| TEXAS INSTRUMENTS INCORPORATED
| Standard Linear and Logic Group
| IBIS Model of SN74LVCC3245A_BIO
| OCTAL BUS TRANSCEIVER WITH ADJUSTABLE OUTPUT VOLTAGE AND 3-STATE OUTPUTS
| This file contains package information for the following:
|  TSSOP 24-pin (PW) package as [Component] LVCC3245A_PW
|  SOP 24-pin (NS) package as [Component] LVCC3245A_NS
|  SOIC 24-pin (DW) package as [Component] LVCC3245A_DW
|  SSOP 24-pin (DB) package as [Component] LVCC3245A_DB
| This device can be powered at the following Vccs:
|  3.3 volt Vcc (B-Port)
|  5 volt Vcc (B-Port)
|  3.3 volt Vcc (A-Port)
|  2.5 volt Vcc (A-Port)
| This file provides unique models under the [Model Selector] for each Vcc.
| For operation at a specific Vcc, select the appropriate model after each
| [Model Selector] keyword.
[IBIS Ver]   3.2
[Comment char]  |_char
[File Name]   sn74lvcc3245a.ibs
[File Rev]   1.1 | b_die
[Date]   October 21, 2002
[Source]   Data created from TI-SPICE simulations at TI-SLL.
[Notes]   The following is an IBIS list for the LVCC3245A.
   Please contact sllibis@ti.com with questions and
   comments concerning SLL IBIS models.
   NON MONOTONIC DATA DUE TO DEVICE CHARECTERISTICS
   - Power-clamp data has been deleted from the input model
   since there is no power-clamp diode.
[Disclaimer] Property of Texas Instruments Incorporated.  Unauthorized
   reproduction and/or distribution is strictly prohibited.
   This product is protected under copyright law.
   Created  2002, (C) Copyright  2002, Texas Instruments
   Incorporated, All Rights Reserved
   UNLESS THERE IS A SIGNED, WRITTEN AGREEMENT TO THE
   CONTRARY, TEXAS INSTRUMENTS (TI) IS PROVIDING THE IBIS
   MODELS  AND WITHOUT ANY WARRANTY, EXPRESSED OR
   IMPLIED.  TI assumes no liability for:
   1) the accuracy of the IBIS models provided to your
   company;
   2) the proper functioning of these IBIS Models in your
   design or for any resulting applications; or
   3) infringement of patents, copyrights or intellectual
   property rights resulting from your use of these IBIS
   models.
   TI provides IBIS Models as a service to our customers.
   You and your company shall not distribute, sell or give
   these models to anyone else without prior written
   permission from TI.
   TI reserves the right to make changes to our products or
   to discontinue any semiconductor product or service
   without notice, and advises our customers to obtain the
   latest version of relevant information to verify, before
   placing orders, that the information being relied on is
   current.
   Please be aware that your receipt and use of the IBIS
   information provided shall serve as acceptance of these
   terms and conditions.  If you do not accept these terms,
   you should return or destroy the IBIS models and any
   other accompanying information immediately.
| Component LVCC3245A_PW 24-pin TSSOP
[Component]   LVCC3245A_PW
[Manufacturer]   Texas Instruments, Inc.
[Package]
|   typ   min   max
R_pkg   3.900e-02   3.000e-02   4.600e-02
L_pkg   2.685e-09   2.367e-09   3.177e-09
C_pkg   3.200e-13   2.520e-13   4.340e-13
[Pin]   signal_name   model_name   R_pin   L_pin   C_pin
1   VCCA   POWER   3.700e-02   3.153e-09   4.340e-13
2   DIR   LVCC3245A_DIR   3.400e-02   2.629e-09   3.410e-13
3   A1   LVCC3245A_AIO   3.200e-02   2.860e-09   3.470e-13
4   A2   LVCC3245A_AIO   4.200e-02   2.741e-09   2.900e-13
5   A3   LVCC3245A_AIO   4.600e-02   2.600e-09   2.620e-13
6   A4   LVCC3245A_AIO   4.300e-02   2.414e-09   2.660e-13
7   A5   LVCC3245A_AIO   4.200e-02   2.367e-09   2.620e-13
8   A6   LVCC3245A_AIO   4.400e-02   2.461e-09   2.520e-13
9   A7   LVCC3245A_AIO   4.200e-02   2.543e-09   2.740e-13
10   A8   LVCC3245A_AIO   3.000e-02   2.616e-09   3.320e-13
11   GND   GND   3.700e-02   2.670e-09   3.460e-13
12   GND   GND   3.900e-02   3.177e-09   4.330e-13
13   GND   GND   3.700e-02   3.111e-09   4.310e-13
14   B8   LVCC3245A_BIO   3.700e-02   2.656e-09   3.450e-13
15   B7   LVCC3245A_BIO   3.100e-02   2.739e-09   3.400e-13
16   B6   LVCC3245A_BIO   4.200e-02   2.649e-09   2.820e-13
17   B5   LVCC3245A_BIO   4.600e-02   2.532e-09   2.570e-13
18   B4   LVCC3245A_BIO   4.400e-02   2.425e-09   2.660e-13
19   B3   LVCC3245A_BIO   4.400e-02   2.425e-09   2.660e-13
20   B2   LVCC3245A_BIO   4.600e-02   2.532e-09   2.570e-13
21   B1   LVCC3245A_BIO   4.200e-02   2.648e-09   2.820e-13
22   OE   LVCC3245A_NOE   3.100e-02   2.738e-09   3.390e-13
23   NC   NC   3.600e-02   2.653e-09   3.440e-13
24   VCCB   POWER   3.700e-02   3.110e-09   4.310e-13
| Component LVCC3245A_NS 24-pin SOP
[Component]   LVCC3245A_NS
[Manufacturer]   Texas Instruments, Inc.
[Package]
|   typ   min   max
R_pkg   4.400e-02   3.800e-02   4.800e-02
L_pkg   3.840e-09   2.545e-09   5.234e-09
C_pkg   5.860e-13   2.740e-13   7.970e-13
[Pin]   signal_name   model_name   R_pin   L_pin   C_pin
1   VCCA   POWER   4.100e-02   5.146e-09   7.650e-13
2   DIR   LVCC3245A_DIR   4.100e-02   4.357e-09   7.490e-13
3   A1   LVCC3245A_AIO   4.000e-02   3.923e-09   6.330e-13
4   A2   LVCC3245A_AIO   4.400e-02   3.412e-09   5.370e-13
5   A3   LVCC3245A_AIO   4.500e-02   3.036e-09   3.970e-13
6   A4   LVCC3245A_AIO   4.500e-02   2.845e-09   4.150e-13
7   A5   LVCC3245A_AIO   4.400e-02   2.843e-09   4.150e-13
8   A6   LVCC3245A_AIO   4.500e-02   3.065e-09   3.990e-13
9   A7   LVCC3245A_AIO   4.500e-02   3.529e-09   5.440e-13
10   A8   LVCC3245A_AIO   4.100e-02   4.013e-09   6.390e-13
11   GND   GND   4.100e-02   4.358e-09   7.460e-13
12   GND   GND   4.400e-02   5.234e-09   7.670e-13
13   GND   GND   3.900e-02   5.181e-09   7.650e-13
14   B8   LVCC3245A_BIO   4.800e-02   4.582e-09   7.640e-13
15   B7   LVCC3245A_BIO   4.100e-02   4.163e-09   6.550e-13
16   B6   LVCC3245A_BIO   4.600e-02   3.613e-09   5.490e-13
17   B5   LVCC3245A_BIO   4.700e-02   3.163e-09   4.060e-13
18   B4   LVCC3245A_BIO   4.700e-02   2.963e-09   4.220e-13
19   B3   LVCC3245A_BIO   4.700e-02   2.919e-09   4.190e-13
20   B2   LVCC3245A_BIO   4.800e-02   3.087e-09   4.870e-13
21   B1   LVCC3245A_BIO   4.600e-02   4.513e-09   7.600e-13
22   OE   LVCC3245A_NOE   4.200e-02   4.505e-09   7.670e-13
23   NC   NC   4.200e-02   5.163e-09   7.970e-13
24   VCCB   POWER   3.800e-02   2.545e-09   2.740e-13
| Component LVCC3245A_DW 24-pin SOIC
[Component]   LVCC3245A_DW
[Manufacturer]   Texas Instruments, Inc.
[Package]
|   typ   min   max
R_pkg   3.700e-02   3.000e-02   4.700e-02
L_pkg   5.146e-09   3.993e-09   6.885e-09
C_pkg   7.580e-13   5.120e-13   1.067e-12
[Pin]   signal_name   model_name   R_pin   L_pin   C_pin
1   VCCA   POWER   3.900e-02   6.885e-09   1.067e-12
2   DIR   LVCC3245A_DIR   4.200e-02   5.950e-09   9.580e-13
3   A1   LVCC3245A_AIO   4.700e-02   5.317e-09   7.910e-13
4   A2   LVCC3245A_AIO   3.100e-02   4.651e-09   6.110e-13
5   A3   LVCC3245A_AIO   3.000e-02   3.993e-09   5.120e-13
6   A4   LVCC3245A_AIO   3.000e-02   4.083e-09   6.110e-13
7   A5   LVCC3245A_AIO   3.000e-02   4.083e-09   6.110e-13
8   A6   LVCC3245A_AIO   3.000e-02   3.993e-09   5.120e-13
9   A7   LVCC3245A_AIO   3.100e-02   4.652e-09   6.110e-13
10   A8   LVCC3245A_AIO   4.700e-02   5.317e-09   7.910e-13
11   GND   GND   4.200e-02   5.950e-09   9.590e-13
12   GND   GND   3.900e-02   6.885e-09   1.067e-12
13   GND   GND   3.900e-02   6.885e-09   1.067e-12
14   B8   LVCC3245A_BIO   4.200e-02   5.950e-09   9.590e-13
15   B7   LVCC3245A_BIO   4.700e-02   5.317e-09   7.910e-13
16   B6   LVCC3245A_BIO   3.100e-02   4.652e-09   6.110e-13
17   B5   LVCC3245A_BIO   3.000e-02   3.993e-09   5.120e-13
18   B4   LVCC3245A_BIO   3.000e-02   4.083e-09   6.100e-13
19   B3   LVCC3245A_BIO   3.000e-02   4.083e-09   6.100e-13
20   B2   LVCC3245A_BIO   3.000e-02   3.993e-09   5.120e-13
21   B1   LVCC3245A_BIO   3.100e-02   4.651e-09   6.110e-13
22   OE   LVCC3245A_NOE   4.700e-02   5.317e-09   7.910e-13
23   NC   NC   4.200e-02   5.950e-09   9.580e-13
24   VCCB   POWER   3.900e-02   6.885e-09   1.067e-12
| Component LVCC3245A_DB 24-pin SSOP
[Component]   LVCC3245A_DB
[Manufacturer]   Texas Instruments, Inc.
[Package]
|   typ   min   max
R_pkg   4.500e-02   4.000e-02   4.900e-02
L_pkg   3.668e-09   3.226e-09   4.415e-09
C_pkg   4.160e-13   3.490e-13   5.070e-13
[Pin]   signal_name   model_name   R_pin   L_pin   C_pin
1   VCCA   POWER   4.200e-02   4.299e-09   5.030e-13
2   DIR   LVCC3245A_DIR   4.000e-02   3.960e-09   4.990e-13
3   A1   LVCC3245A_AIO   4.200e-02   3.775e-09   4.170e-13
4   A2   LVCC3245A_AIO   4.700e-02   3.487e-09   3.690e-13
5   A3   LVCC3245A_AIO   4.600e-02   3.347e-09   3.520e-13
6   A4   LVCC3245A_AIO   4.900e-02   3.352e-09   3.710e-13
7   A5   LVCC3245A_AIO   4.600e-02   3.226e-09   3.630e-13
8   A6   LVCC3245A_AIO   4.700e-02   3.289e-09   3.490e-13
9   A7   LVCC3245A_AIO   4.700e-02   3.347e-09   3.610e-13
10   A8   LVCC3245A_AIO   4.100e-02   3.576e-09   4.090e-13
11   GND   GND   4.100e-02   3.995e-09   5.030e-13
12   GND   GND   4.500e-02   4.415e-09   5.070e-13
13   GND   GND   4.300e-02   4.337e-09   5.060e-13
14   B8   LVCC3245A_BIO   4.200e-02   4.003e-09   5.040e-13
15   B7   LVCC3245A_BIO   4.100e-02   3.686e-09   4.100e-13
16   B6   LVCC3245A_BIO   4.800e-02   3.355e-09   3.490e-13
17   B5   LVCC3245A_BIO   4.700e-02   3.301e-09   3.530e-13
18   B4   LVCC3245A_BIO   4.800e-02   3.268e-09   3.660e-13
19   B3   LVCC3245A_BIO   4.800e-02   3.269e-09   3.660e-13
20   B2   LVCC3245A_BIO   4.700e-02   3.314e-09   3.490e-13
21   B1   LVCC3245A_BIO   4.800e-02   3.399e-09   3.550e-13
22   OE   LVCC3245A_NOE   4.100e-02   3.688e-09   4.120e-13
23   NC   NC   4.200e-02   4.003e-09   5.040e-13
24   VCCB   POWER   4.300e-02   4.347e-09   5.050e-13
| Model LVCC3245A_NOE
[Model Selector]   LVCC3245A_NOE
LVCC3245A_NOE_33   3.3 volt Vcc
LVCC3245A_NOE_25   2.5 volt Vcc
| Model LVCC3245A_DIR
[Model Selector]   LVCC3245A_DIR
LVCC3245A_DIR_33   3.3 volt Vcc
LVCC3245A_DIR_25   2.5 volt Vcc
| Model LVCC3245A_AIO
[Model Selector]   LVCC3245A_AIO
LVCC3245A_AIO_33   3.3 volt Vcc
LVCC3245A_AIO_25   2.5 volt Vcc
| Model LVCC3245A_BIO
[Model Selector]   LVCC3245A_BIO
LVCC3245A_BIO_33   3.3 volt Vcc
LVCC3245A_BIO_50   5 volt Vcc
| Models and submodels in the file (8): LVCC3245A_BIO_33 (I/O), LVCC3245A_BIO_50 (I/O), LVCC3245A_NOE_33 (Input), LVCC3245A_NOE_25 (Input), LVCC3245A_DIR_33 (Input), LVCC3245A_DIR_25 (Input), LVCC3245A_AIO_33 (I/O), LVCC3245A_AIO_25 (I/O)
